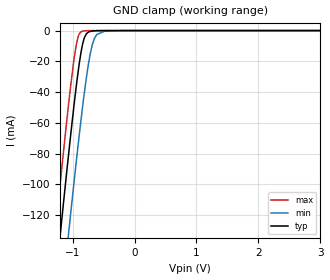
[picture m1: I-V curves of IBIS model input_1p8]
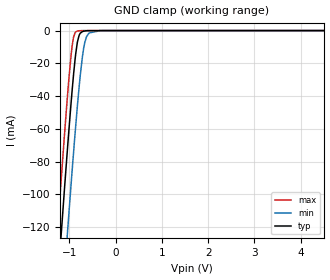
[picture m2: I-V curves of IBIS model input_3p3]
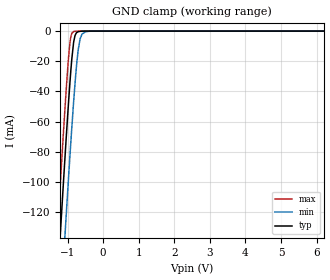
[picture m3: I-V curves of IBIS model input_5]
|Texas Instruments Incorporated
| 16-Bit,500-kSPS,4- and 8- Channel,Single-Supply,SAR ADCs with Programmable,
| Bipolar Input Range
| Marketing part#   Digital Voltage Range   Package-type   #pins
| ADS8688DBT   1.65V-5.25V   TSSOP   38
[IBIS Ver]   4.1
[File name]   ads8688.ibs
[File Rev]   1.0
[Date]   3/12/2014
[Source]
| Texas Instruments Incorporated.
| Analog-eLab Design Center, HPA
| 12500 TI Blvd
| Dallas, TX -75243
[Notes]   Revision History:
| Rev 1.0: 3/12/2014
| - Initial version of the model
| - Model generated from simulations in TISPICE
| - Model matched to SPICE simulation
| - C_comp although listed in numerical order of value are
|   obtained from varying PVT conditions. For PVT conditions for
|   each specific value refer the buffer description under
|   respective [Model]. IBIS model user is responsible for using
|   appropriate C_comp to simulate for Signal Integrity.
[Disclaimer]
| This model is designed as an aid for customers of Texas Instruments.
| TI and its licensors and suppliers make no warranties, either expressed
| or implied, with respect to this  model, including the warranties of
| merchantability or fitness for a particular purpose. The model is
| provided solely on an "as is" basis. The entire risk as to its quality
| and performance is with the customer.
[Copyright]
(C) Copyright 2014 Texas Instruments Incorporated.All rights reserved.
|   ADS8688DBT
[Component]   ADS8688DBT
[Manufacturer]   TI
[Package]   |38 TSSOP  -  DBT package
|   typ   min   max
R_pkg   0.01   0.008   0.12
L_pkg   1.0nH   0.8nH   1.2nH
C_pkg   0.2pF   0.16pF   0.24pF
[Pin]  signal_name   model_name   R_pin   L_pin   C_pin
1   SDI   INPUT   NA   NA   NA
2   RSTZ/PDZ   INPUT   NA   NA   NA
3   DAISY   INPUT   NA   NA   NA
4   REFSELZ   INPUT   NA   NA   NA
5   REFIO   NC   NA   NA   NA
6   REFGND   GND   NA   NA   NA
7   REFCAP   NC   NA   NA   NA
8   AGND   GND   NA   NA   NA
9   AVDD   POWER   NA   NA   NA
10   AUX_IN   NC   NA   NA   NA
11   AUX_GND   NC   NA   NA   NA
12   AIN_6P   NC   NA   NA   NA
13   AIN_6GND   NC   NA   NA   NA
14   AIN_7P   NC   NA   NA   NA
15   AIN_7GND   NC   NA   NA   NA
16   AIN_0P   NC   NA   NA   NA
17   AIN_0GND   NC   NA   NA   NA
18   AIN_1P   NC   NA   NA   NA
19   AIN_1GND   NC   NA   NA   NA
20   AIN2_GND   NC   NA   NA   NA
21   AIN_2P   NC   NA   NA   NA
22   AIN_3GND   NC   NA   NA   NA
23   AIN_3P   NC   NA   NA   NA
24   AIN_4GND   NC   NA   NA   NA
25   AIN_4P   NC   NA   NA   NA
26   AIN_5GND   NC   NA   NA   NA
27   AIN_5P   NC   NA   NA   NA
28   AGND   GND   NA   NA   NA
29   AGND   GND   NA   NA   NA
30   AVDD   POWER   NA   NA   NA
31   AGND   GND   NA   NA   NA
32   AGND   GND   NA   NA   NA
33   DGND   GND   NA   NA   NA
34   DVDD   POWER   NA   NA   NA
35   DNC   NC   NA   NA   NA
36   SDO   TRISTATE   NA   NA   NA
37   SCLK   INPUT   NA   NA   NA
38   CSZ   INPUT   NA   NA   NA
|   Model Selectors
[Model Selector] INPUT
input_1p8   1.8V  digital input
input_3p3   3.3V  digital input
input_5   5.0V  digital input
[Model Selector] TRISTATE
tristate_1p8   1.8V  digital 3-state
tristate_3p3   3.3V  digital 3-state
tristate_5   5.0V  digital 3-state
| Models and submodels in the file (6): input_1p8 (Input), input_3p3 (Input), input_5 (Input), tristate_1p8 (3-state), tristate_3p3 (3-state), tristate_5 (3-state)
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|   input_1p8 Model
[Model]   input_1p8
Model_type   Input
Vinl = 0.36
Vinh = 1.44
|   typ   min   max
|   (nom PVT)   (fast PVT)   (slow PVT)
C_comp   3.865e-13   3.082e-13   4.643e-13
[Model spec]
|subparameter
Vinl   0.36   0.33   0.39
Vinh   1.44   1.32   1.56
| Where nom  PVT is Nominal Process, 1.8V, 27C
|   Fast PVT is Strong Process,  1.95V, -40C
|   Slow PVT is Weak Process,   1.65V, 125C
[Voltage Range]   1.8   1.65   1.95
|Junction Temperature
[Temperature Range]   27   125   -40
[Power Clamp Reference]   1.8   1.65   1.95
[GND Clamp Reference]   0   0   0
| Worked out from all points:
|   GND clamp passes 1 mA (typ) near -0.74 V on its own axis
[GND Clamp]
|   Voltage   I(typ)   I(min)   I(max)
-1.8V     -379.9mA   -431.2mA   -347mA
-1.386V   -208.3mA   -260.4mA   -174.8mA
-1.182V   -126.1mA   -178.2mA   -92.69mA
-1.089V   -89.99mA   -141.7mA   -57.08mA
-1.048V   -74.35mA   -125.7mA   -42mA
-938.1mV  -35.63mA   -84.56mA   -8.858mA
-862mV    -13.89mA   -57.64mA   -796.7uA
-779.4mV  -2.256mA   -31.39mA   -88.53uA
-682.9mV  -321.8uA   -9.377mA   -6.522uA
-608.7mV  -78.53uA   -2.561mA   -592.7nA
-488.3mV  -4.259uA   -475.2uA   0A
3.6V      0A         0A         0A
[POWER Clamp]
|   Voltage   I(typ)   I(min)   I(max)
-1.8V     0A         0A         0A
0V        0A         0A         0A
3.6V      0A         0A         0A
|   input_3p3 Model
[Model]   input_3p3
Model_type   Input
Vinl = 0.99
Vinh = 2.31
|   typ   min   max
|   (nom PVT)   (fast PVT)   (slow PVT)
C_comp   3.611e-13   2.944e-13   4.265e-13
[Model spec]
|subparameter
Vinl   0.99   0.9   1.08
Vinh   2.31   2.1   2.52
| Where nom  PVT is Nominal Process, 3.3V, 27C
|   Fast PVT is Strong Process,  3.6V, -40C
|   Slow PVT is Weak Process,   3V, 125C
[Voltage Range]   3.3   3   3.6
|Junction Temperature
[Temperature Range]   27   125   -40
[Power Clamp Reference]   3.3   3   3.6
[GND Clamp Reference]   0   0   0
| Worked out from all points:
|   GND clamp passes 1 mA (typ) near -0.74 V on its own axis
[GND Clamp]
|   Voltage   I(typ)   I(min)   I(max)
-3.3V     -1.016A    -1.064A    -984.6mA
-1.633V   -310.3mA   -362mA     -277.2mA
-1.234V   -146.7mA   -198.9mA   -113.2mA
-1.198V   -132.5mA   -184.6mA   -99.01mA
-1.104V   -95.75mA   -147.6mA   -62.7mA
-1.038V   -70.78mA   -122mA     -38.62mA
-937.2mV  -35.34mA   -84.23mA   -8.673mA
-831mV    -7.706mA   -47.29mA   -316.6uA
-765.6mV  -1.619mA   -27.5mA    -63.18uA
-689.7mV  -362.1uA   -10.45mA   -7.983uA
-573mV    -35.69uA   -1.45mA    -167.5nA
6.6V      0A         0A         0A
[POWER Clamp]
|   Voltage   I(typ)   I(min)   I(max)
-3.3V     0A         0A         0A
0V        0A         0A         0A
6.6V      0A         0A         0A
|   input_5 Model
[Model]   input_5
Model_type   Input
Vinl = 1.5
Vinh = 3.5
|   typ   min   max
|   (nom PVT)   (fast PVT)   (slow PVT)
C_comp   3.420e-13   2.827e-13   4.012e-13
[Model spec]
|subparameter
Vinl   1.5   1.425   1.575
Vinh   3.5   3.325   3.675
| Where nom  PVT is Nominal Process, 5V, 27C
|   Fast PVT is Strong Process,  5.25V, -40C
|   Slow PVT is Weak Process,   4.75V, 125C
[Voltage Range]   5   4.75   5.25
|Junction Temperature
[Temperature Range]   27   125   -40
[Power Clamp Reference]   5   4.75   5.25
[GND Clamp Reference]   0   0   0
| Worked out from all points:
|   GND clamp passes 1 mA (typ) near -0.74 V on its own axis
[GND Clamp]
|   Voltage   I(typ)   I(min)   I(max)
-5V       -1.743A    -1.788A    -1.713A
-1.3V     -173.4mA   -225.6mA   -139.9mA
-1.278V   -164.4mA   -216.6mA   -130.9mA
-1.186V   -127.7mA   -179.8mA   -94.23mA
-1.115V   -99.99mA   -151.9mA   -66.85mA
-1.042V   -72.08mA   -123.4mA   -39.85mA
-938.7mV  -35.84mA   -84.8mA    -9.006mA
-831.5mV  -7.792mA   -47.46mA   -320.7uA
-745mV    -1.022mA   -22.08mA   -37.54uA
-649mV    -174.9uA   -5.226mA   -2.273uA
-463.7mV  -2.19uA    -349.6uA   0A
10V       0A         0A         0A
[POWER Clamp]
|   Voltage   I(typ)   I(min)   I(max)
-5V       0A         0A         0A
0V        0A         0A         0A
10V       0A         0A         0A
